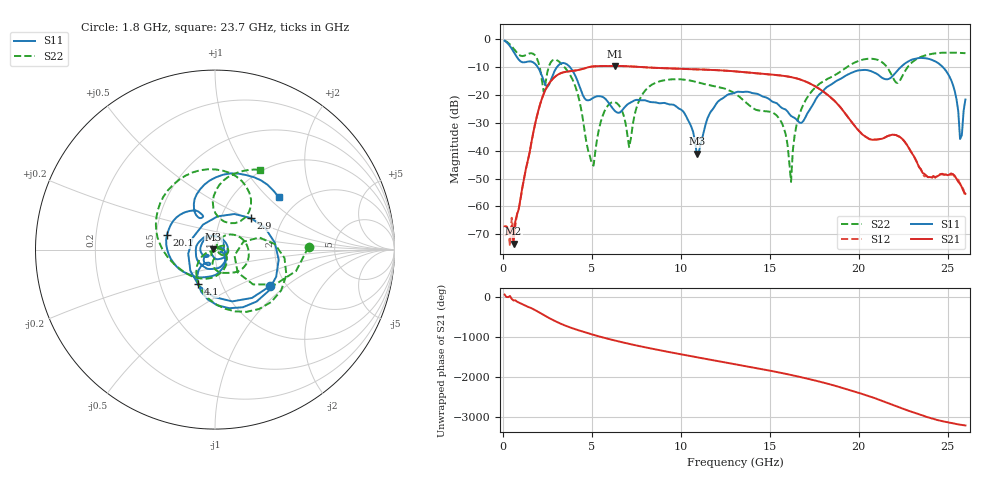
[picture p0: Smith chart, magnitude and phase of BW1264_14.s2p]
!Keysight Technologies,N5245B,MY57181159,A.13.60.06
!Date: Friday, December 18, 2020 23:52:38
!Correction: S11(Full 2 Port(1,2))
!S21(Full 2 Port(1,2))
!S12(Full 2 Port(1,2))
!S22(Full 2 Port(1,2))
!S2P File: Measurements: S11, S21, S12, S22:
# Hz S  dB  R 50
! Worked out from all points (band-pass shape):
!   260 points, 100 MHz to 26 GHz, reference 50 ohm
!   highest |S21| = -9.55 dB at 6.3 GHz (marker M1); lowest = -73.4 dB at 600 MHz (marker M2)
!   |S21| within 3 dB of the highest: 3.13 GHz to 14.93 GHz (11.8 GHz wide, 131 % of centre)
!   lowest |S11| = -41.1 dB at 10.9 GHz (marker M3), VSWR 1.02, Z = 49.1 + j0.186 ohm
!   |S11| at or under -10 dB: 1.964 GHz to 3.038 GHz (1.074 GHz wide, 42.9 % of centre); 3.776 GHz to 22.36 GHz (18.58 GHz wide, 142 % of centre); 24.73 GHz to end of sweep
!   |S22| runs from -51.2 to -0.4 dB; largest |S21 - S12| = 0.00069
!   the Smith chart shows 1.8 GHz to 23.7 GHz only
!   S11 on the Smith chart (normalised r, x): 1.8 GHz: 1.65, -0.78; 2.9 GHz: 1.39, +0.52; 4.1 GHz: 0.77, -0.31; 20.1 GHz: 0.57, +0.10; 23.7 GHz: 1.57, +1.17
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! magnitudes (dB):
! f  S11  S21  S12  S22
! 100 MHz  -0.5  -67.2  -70.4  -0.4
! 600 MHz  -4.4  -73.4  -68.9  -3.3
! 1.8 GHz  -8.7  -30.7  -30.8  -5.7
! 2.3 GHz  -14.8  -19.5  -19.5  -18.9
! 2.9 GHz  -11.5  -13.6  -13.6  -7.3
! 4.1 GHz  -13.4  -11.2  -11.2  -17.3
! 4.5 GHz  -20.1  -10.6  -10.6  -28.7
! 5.1 GHz  -20.9  -9.7  -9.7  -45.3
! 6.3 GHz  -25.7  -9.6  -9.6  -22.6
! 7.1 GHz  -23.0  -9.7  -9.7  -38.7
! 8.8 GHz  -23.0  -10.3  -10.3  -15.1
! 10.9 GHz  -41.1  -10.8  -10.8  -15.4
! 13.1 GHz  -19.0  -11.5  -11.5  -19.6
! 15.6 GHz  -24.2  -13.0  -13.0  -29.1
! 16.2 GHz  -27.5  -13.6  -13.6  -51.2
! 17.4 GHz  -23.7  -16.3  -16.3  -18.4
! 20.1 GHz  -11.1  -33.4  -33.4  -7.5
! 21.7 GHz  -14.2  -34.6  -34.6  -11.0
! 23.7 GHz  -6.7  -48.3  -49.2  -5.8
! 25.2 GHz  -14.6  -48.1  -48.6  -4.8
! 25.7 GHz  -35.8  -51.8  -52.0  -4.9
! 26 GHz  -21.6  -55.5  -56.7  -5.0
